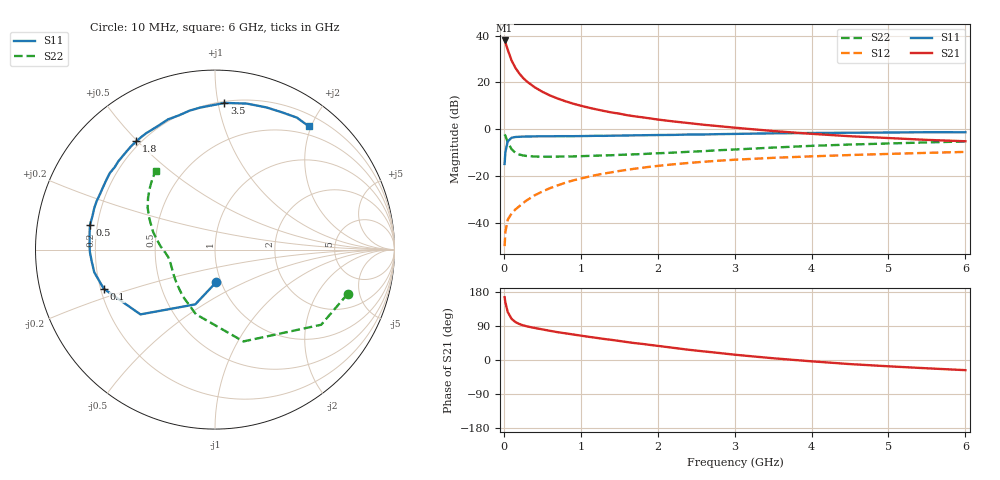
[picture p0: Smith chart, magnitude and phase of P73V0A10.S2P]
! SIEMENS Small Signal Semiconductors
! BFP196
! Si NPN RF Bipolar Junction Transistor in SOT143
! VCE = 3 V  IC = 100 mA
! Common Emitter S-Parameters:  May  1996
# GHz  S  MA  R  50
!  f  S11  S21  S12  S22
! GHz  MAG  ANG  MAG  ANG  MAG  ANG  MAG  ANG
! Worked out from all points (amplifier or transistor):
!   36 points, 10 MHz to 6 GHz, reference 50 ohm
!   highest |S21| = 37.9 dB at 10 MHz (marker M1)
!   |S21| within 3 dB of that: start of sweep to 41.22 MHz
!   unconditionally stable (mu >= 1): 291.1 MHz to 5.068 GHz
!   at 250 MHz: K = 0.97, MSG = 26.7 dB, |S12| = -31.5 dB
!   at 1.4 GHz: K = 1.10, MAG = 10.9 dB, |S12| = -18.4 dB
!   at 6 GHz: K = 0.99, MSG = 2.3 dB, |S12| = -9.7 dB
!   S11 on the Smith chart (normalised r, x): 10 MHz: 0.95, -0.36; 100 MHz: 0.21, -0.16; 500 MHz: 0.17, +0.09; 1.8 GHz: 0.18, +0.50; 3.5 GHz: 0.21, +1.04; 6 GHz: 0.36, +1.96
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0.01  0.1819 -87.9  78.52 165.7  0.0032 77.6  0.7797 -18.4
0.02  0.3242 -109.8  71.51 152.2  0.0064 66.3  0.7248 -35.3
0.05  0.5503 -139.0  50.09 126.9  0.0117 54.9  0.5356 -72.8
0.1  0.657 -160.6  29.57 108.7  0.0159 52.7  0.3755 -106.5
0.15  0.6845 -169.4  20.46 100.2  0.0194 55.2  0.3157 -124.7
0.2  0.6901 -174.6  15.57 95.1  0.0227 58.5  0.2894 -135.9
0.25  0.6972 -178.9  12.46 91.5  0.0266 61.6  0.276 -144.0
0.3  0.6991 178.2  10.44 88.8  0.0306 64.1  0.269 -149.2
0.4  0.7044 172.8  7.892 84.6  0.0389 66.2  0.2617 -156.7
0.5  0.7098 168.9  6.311 80.8  0.0469 67.1  0.2597 -161.4
0.6  0.7076 164.9  5.263 77.0  0.0554 66.8  0.2593 -164.6
0.7  0.7117 160.8  4.525 73.4  0.0635 66.5  0.2606 -167.1
0.9  0.7116 154.1  3.522 67.4  0.081 64.7  0.2635 -170.9
1.1  0.7192 147.3  2.897 61.3  0.097 62.6  0.2702 -173.6
1.4  0.7293 137.7  2.285 53.1  0.1206 58.2  0.2792 -177.1
1.8  0.7456 126.0  1.798 42.5  0.1508 52.0  0.2954 178.3
2.2  0.7576 115.4  1.472 32.2  0.1783 45.8  0.317 173.0
2.8  0.787 100.4  1.162 18.5  0.2136 36.6  0.3575 164.3
3.5  0.8189 86.3  0.917 4.6  0.2456 26.4  0.4063 154.4
4.5  0.8425 70.1  0.71 -10.8  0.2818 14.2  0.4719 142.2
5.5  0.8654 58.2  0.593 -21.9  0.3136 3.3  0.524 132.0
6  0.8632 52.8  0.555 -26.8  0.3286 -2.4  0.5491 127.0
